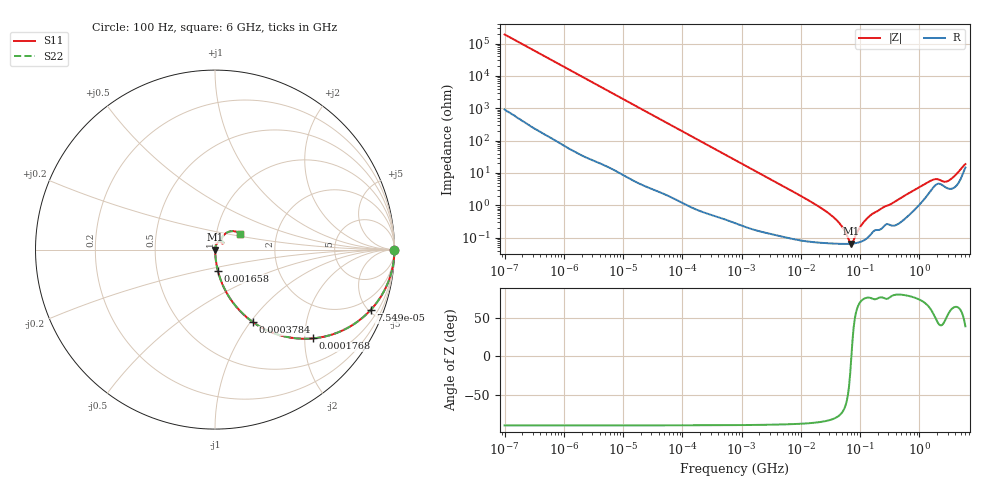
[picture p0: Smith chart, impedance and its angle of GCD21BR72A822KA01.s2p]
!Murata Part Number: GCD21BR72A822KA01
!These Parameters are Measured in Series Mode Connection
!Data Generated on Jan 08, 2026
!  o--ll--o
!Port1  Port2
!  o------o
!Operation Temp=25[degC], DC Bias Voltage=0[V]
!Freq. Start=100[Hz] Stop=6[GHz] 401[Steps]
# Hz S RI R 50
!Freq.(Hz) S11(Real) S11(Imag) S21(Real) S21(Imag) S12(Real) S12(Imag) S22(Real) S22(Imag)
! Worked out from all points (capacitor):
!   401 points, 100 Hz to 6 GHz, reference 50 ohm
!   read as one part in series: C = 8.35 nF near 109 Hz
!   lowest |Z| = 65.7 mohm at 71.29 MHz (marker M1)
!   series resonance near 71.45 MHz, so ESL is about 590 pH
!   S11 on the Smith chart (normalised r, x): 100 Hz: open; 75.5 kHz: 1.03, -5.14; 176.8 kHz: 1.01, -2.20; 378.4 kHz: 1.01, -1.03; 1.658 MHz: 1.00, -0.24; 6 GHz: 1.29, +0.24
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100  1 -0.000525  2.8e-06 0.000525  2.8e-06 0.000525  1 -0.000525
2008  0.9999 -0.0105  0.000148 0.0105  0.000148 0.0105  0.9999 -0.0105
12592  0.9955 -0.065  0.00454 0.065  0.00454 0.065  0.9955 -0.065
40335  0.9573 -0.1994  0.0427 0.1994  0.0427 0.1994  0.9573 -0.1994
75495  0.8669 -0.3367  0.1331 0.3367  0.1331 0.3367  0.8669 -0.3367
176758  0.5472 -0.4945  0.4528 0.4945  0.4528 0.4945  0.5472 -0.4945
378399  0.2119 -0.4043  0.7881 0.4043  0.7881 0.4043  0.2119 -0.4043
774597  0.0624 -0.2363  0.9376 0.2363  0.9376 0.2363  0.0624 -0.2363
1658239  0.0155 -0.1165  0.9845 0.1165  0.9845 0.1165  0.0155 -0.1165
1.555665e7  0.000887 -0.0122  0.9991 0.0122  0.9991 0.0122  0.000887 -0.0122
3.983537e7  0.000666 -0.0035  0.9993 0.0035  0.9993 0.0035  0.000666 -0.0035
4.983056e7  0.00065 -0.0021  0.9994 0.0021  0.9994 0.0021  0.00065 -0.0021
6.518806e7  0.000649 -0.000527  0.9994 0.000527  0.9994 0.000527  0.000649 -0.000527
7.129496e7  0.000656 -1.25e-05  0.9993 1.25e-05  0.9993 1.25e-05  0.000656 -1.25e-05
7.797396e7  0.000668 0.000505  0.9993 -0.000505  0.9993 -0.000505  0.000668 0.000505
1.020051e8  0.000752 0.00212  0.9992 -0.00212  0.9992 -0.00212  0.000752 0.00212
1.334425e8  0.00101 0.00394  0.999 -0.00394  0.999 -0.00394  0.00101 0.00394
1.669249e8  0.00158 0.00546  0.9984 -0.00546  0.9984 -0.00546  0.00158 0.00546
3.124326e8  0.00263 0.01  0.9974 -0.01  0.9974 -0.01  0.00263 0.01
1.637704e9  0.0332 0.0479  0.9668 -0.0479  0.9668 -0.0479  0.0332 0.0479
3.065283e9  0.034 0.0433  0.966 -0.0433  0.966 -0.0433  0.034 0.0433
6e9  0.1375 0.0887  0.8625 -0.0887  0.8625 -0.0887  0.1375 0.0887
